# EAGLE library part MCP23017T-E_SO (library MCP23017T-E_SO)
Interface - I/O Expanders 16bit Input/Output Exp I2C interface Source: Datasheet
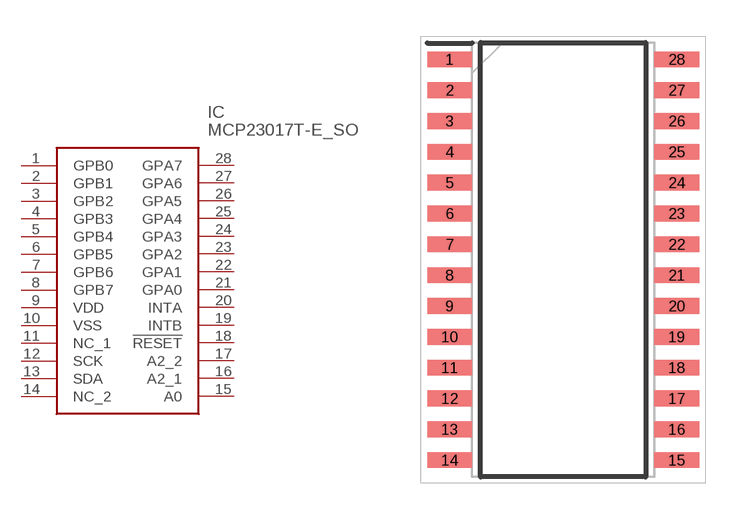
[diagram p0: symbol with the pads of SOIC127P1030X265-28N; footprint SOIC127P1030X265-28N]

Designator prefix IC

## MCP23017T-E_SO (Description: Interface - I/O Expanders 16bit Input/Output Exp I2C interface; Height: 2.65mm; Manufacturer_Name: Microchip; Manufacturer_Part_Number: MCP23017T-E/SO; Mouser_Part_Number: 579-MCP23017T-E/SO; Mouser_Price-Stock: https://www.mouser.co.uk/ProductDetail/Microchip-Technology/MCP23017T-E-SO?qs=usxtMOJb1RylPfT%252BJtgE3Q%3D%3D)  [SOIC127P1030X265-28N]
1  GPB0
2  GPB1
3  GPB2
4  GPB3
5  GPB4
6  GPB5
7  GPB6
8  GPB7
9  VDD
10  VSS
11  NC_1
12  SCK
13  SDA
14  NC_2
15  A0
16  A2_1
17  A2_2
18  !RESET
19  INTB
20  INTA
21  GPA0
22  GPA1
23  GPA2
24  GPA3
25  GPA4
26  GPA5
27  GPA6
28  GPA7

## Footprint SOIC127P1030X265-28N (pad centres in mm)
(SO)28-Lead(SOIC)
smd 1.85 x 0.65: 1 -4.675,8.255; 2 -4.675,6.985; 3 -4.675,5.715; 4 -4.675,4.445; 5 -4.675,3.175; 6 -4.675,1.905; 7 -4.675,0.635; 8 -4.675,-0.635; 9 -4.675,-1.905; 10 -4.675,-3.175; 11 -4.675,-4.445; 12 -4.675,-5.715; 13 -4.675,-6.985; 14 -4.675,-8.255; 15 4.675,-8.255; 16 4.675,-6.985; 17 4.675,-5.715; 18 4.675,-4.445; 19 4.675,-3.175; 20 4.675,-1.905; 21 4.675,-0.635; 22 4.675,0.635; 23 4.675,1.905; 24 4.675,3.175; 25 4.675,4.445; 26 4.675,5.715; 27 4.675,6.985; 28 4.675,8.255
